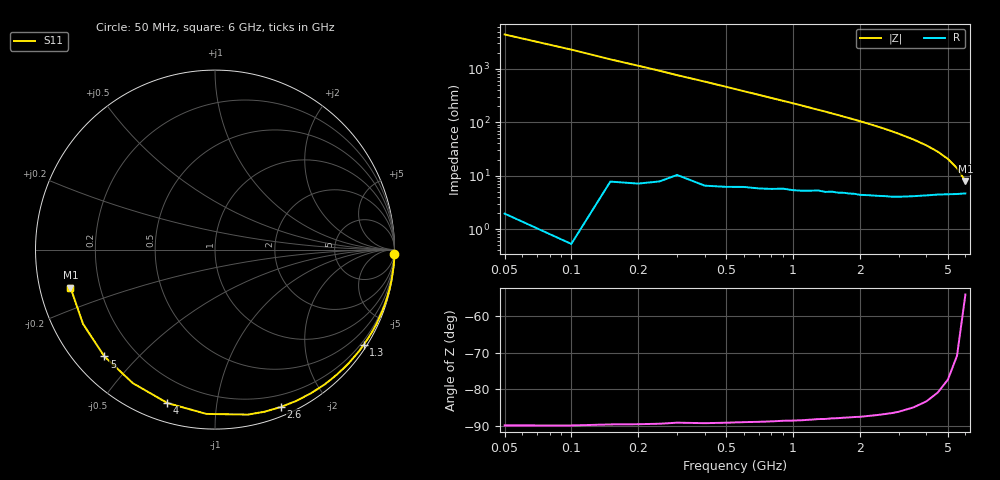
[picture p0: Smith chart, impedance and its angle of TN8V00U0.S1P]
! SIEMENS Discrete & RF Semiconductors
! BAS70-07W
! Si Schottky Diode in SOT343
! VR = 8 V
! S-Parameters:  February  1997
# GHz  S  MA  R  50
!  f  S11
! GHz  MAG  ANG
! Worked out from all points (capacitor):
!   34 points, 50 MHz to 6 GHz, reference 50 ohm
!   read as one part to ground: C = 704 fF near 50 MHz
!   lowest |Z| = 7.9 ohm at 6 GHz (marker M1)
!   S11 on the Smith chart (normalised r, x): 50 MHz: 0, -88; 1.3 GHz: 0.11, -3.42; 2.6 GHz: 0.08, -1.50; 4 GHz: 0.09, -0.73; 5 GHz: 0.09, -0.40; 6 GHz: 0.09, -0.13
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0.05  1 -1.3
0.2  0.9995 -5.0
0.4  0.9981 -9.9
0.5  0.9971 -12.4
0.6  0.9959 -14.9
0.7  0.9947 -17.4
0.8  0.9933 -19.9
1  0.9901 -24.9
1.1  0.9884 -27.4
1.2  0.9861 -30.0
1.3  0.9835 -32.6
1.4  0.9821 -35.1
1.6  0.9775 -40.3
1.7  0.9747 -43.0
1.8  0.9726 -45.6
1.9  0.97 -48.2
2  0.9682 -50.9
2.2  0.9624 -56.3
2.4  0.9567 -61.8
2.6  0.9505 -67.3
2.8  0.9446 -73.0
3  0.9373 -78.7
3.5  0.9168 -93.0
4  0.8951 -107.2
4.5  0.8737 -121.6
5  0.8569 -136.0
5.5  0.8439 -150.6
6  0.8327 -165.3
